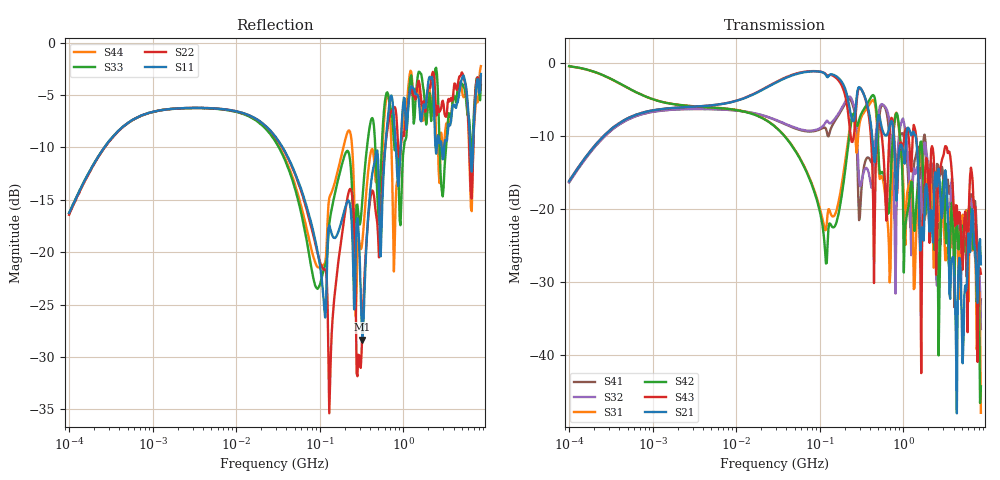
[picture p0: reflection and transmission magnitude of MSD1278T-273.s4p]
# MHz S MA R 50
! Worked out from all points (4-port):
!   498 points, 100 kHz to 8.5 GHz, reference 50 ohm
!   strongest paths, dB at 100 kHz, 1.698 MHz, 29.49 MHz, 500.7 MHz, 8.5 GHz:
!     S21: -16.1, -6.1, -2.7, -7.3, -27.6
!     S43: -16.1, -6.1, -2.6, -7.6, -28.8
!     S42: -0.4, -5.6, -8.7, -11.0, -44.3
!     S31: -0.4, -5.6, -8.7, -12.1, -47.9
!     S32: -16.3, -6.4, -7.7, -7.4, -36.4
!     S41: -16.3, -6.4, -7.8, -10.2, -32.3
!   lowest |S11| = -28.3 dB at 324.4 MHz (marker M1), VSWR 1.08, Z = 46.4 - j0.557 ohm
!   |S11| at or under -10 dB: 35.93 MHz to 609.5 MHz (573.6 MHz wide, 178 % of centre); 2.883 GHz to 3.094 GHz (211.4 MHz wide, 7.07 % of centre); 6.343 GHz to 6.846 GHz (503 MHz wide, 7.63 % of centre)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
0.1  0.154 69.7  0.1559 70.4  0.9533 -8.9  0.1528 -110.1
     0.1559 70.4  0.1508 70.2  0.153 -110.0  0.9547 -8.9
     0.9533 -8.9  0.153 -110.0  0.1534 70.2  0.156 70.3
     0.1528 -110.1  0.9547 -8.9  0.156 70.3  0.1533 70.6
118.7648  0.05353 3.0  0.8287 -31.0  0.07239 -121.5  0.3556 48.0
          0.8287 -31.0  0.08109 -66.0  0.397 51.2  0.04247 -125.4
          0.07239 -121.5  0.397 51.2  0.08835 19.7  0.8394 -36.6
          0.3556 48.0  0.04247 -125.4  0.8394 -36.6  0.09487 29.5
324.4107  0.03831 -171.0  0.6432 -71.5  0.4429 8.4  0.1632 -8.3
          0.6432 -71.5  0.04318 133.9  0.1643 -33.0  0.4662 10.7
          0.4429 8.4  0.1643 -33.0  0.179 31.1  0.6426 -81.8
          0.1632 -8.3  0.4662 10.7  0.6426 -81.8  0.1128 -0.1
2365.873  0.413 134.5  0.1518 149.9  0.04069 123.0  0.05757 120.5
          0.1518 149.9  0.6581 152.9  0.1136 74.2  0.05272 89.1
          0.04069 123.0  0.1136 74.2  0.6931 172.5  0.1662 88.1
          0.05757 120.5  0.05272 89.1  0.1662 88.1  0.611 145.5
3568.796  0.4005 21.8  0.02637 -127.0  0.08739 35.5  0.1271 -7.4
          0.02637 -127.0  0.5227 5.4  0.06776 32.2  0.03902 24.1
          0.08739 35.5  0.06776 32.2  0.4581 18.4  0.2475 -23.5
          0.1271 -7.4  0.03902 24.1  0.2475 -23.5  0.4148 17.0
6462.473  0.2693 158.1  0.07149 76.8  0.09354 69.2  0.1267 100.8
          0.07149 76.8  0.1895 156.7  0.1002 90.4  0.09299 70.3
          0.09354 69.2  0.1002 90.4  0.3153 134.6  0.1926 43.7
          0.1267 100.8  0.09299 70.3  0.1926 43.7  0.1626 175.2
8500  0.7079 -31.0  0.04191 -115.5  0.004034 139.3  0.02417 -109.6
      0.04191 -115.5  0.6909 -39.1  0.01512 40.6  0.006118 -55.3
      0.004034 139.3  0.01512 40.6  0.6276 -32.6  0.03616 -138.8
      0.02417 -109.6  0.006118 -55.3  0.03616 -138.8  0.7713 -39.4
